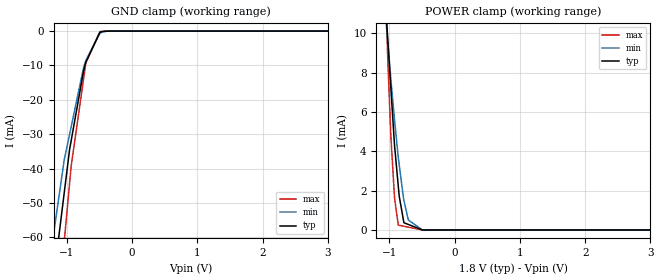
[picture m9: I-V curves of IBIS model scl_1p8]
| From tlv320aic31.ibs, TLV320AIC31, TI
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|   scl_1p8 Model
[Model]   scl_1p8
Model_type   Input
Vinl = 0.54
Vinh = 1.26
|   typ   min   max
|   (nom PVT)   (fast PVT)   (slow PVT)
|C_comp from frequency sweep method (F=400KHz)
|Average
|C_comp   2.312e-11   2.229e-11   2.341e-11
|C_comp from LC tank measurement(L=1nH)
|Average
|Resonant Frequency(Hz)   2.030e+09   2.040e+09   2.020e+09
C_comp   6.153e-12   6.093e-12   6.214e-12
| Where nom  PVT is Nominal Process, 1.8V, 26C
|   Fast PVT is Strong Process,  1.98V, -40C
|   Slow PVT is Weak Process,   1.62V, 86C
[Model Spec]
|Subparameter   typ   min   max
Vinl   0.54   0.486   0.594
Vinh   1.26   1.134   1.386
[Voltage Range]   1.8   1.62   1.98
|Ambient Temperature   25   85   -40
|Junction Temperature
[Temperature Range]   26   86   -40
[Power Clamp Reference]   1.8   1.62   1.98
[GND Clamp Reference]   0   0   0
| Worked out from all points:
|   GND clamp passes 1 mA (typ) near -0.51 V on its own axis
|   POWER clamp passes 1 mA (typ) near -0.81 V on its own axis
[GND Clamp]
|   Voltage   I(typ)   I(min)   I(max)
-1.8V     -330.6mA   -175mA     -470.5mA
-1.202V   -71.76mA   -58.79mA   -94.27mA
-1.04V    -46.94mA   -37.39mA   -61.03mA
-957.6mV  -34.34mA   -29.93mA   -44.11mA
-932.6mV  -31.68mA   -27.67mA   -39.04mA
-745.2mV  -11.71mA   -10.72mA   -14.06mA
-712.8mV  -9.192mA   -8.64mA    -9.745mA
-704.9mV  -8.873mA   -8.35mA    -9.025mA
-495mV    -409.6uA   -657.6uA   -178.1uA
-424.4mV  -70.4uA    -146.2uA   -21.27uA
-306.2mV  -3.142uA   -7.691uA   -346.8nA
3.6V      0A         0A         0A
[POWER Clamp]
|   Voltage   I(typ)   I(min)   I(max)
-1.8V     58.58mA    42.75mA    96.1mA
-1.073V   12.51mA    11.5mA     13.37mA
-1.033V   10.12mA    9.9mA      9.534mA
-1.022V   9.52mA     9.438mA    8.427mA
-976.1mV  7.154mA    7.627mA    4.701mA
-920.7mV  4.294mA    5.584mA    1.615mA
-863.3mV  2.217mA    3.671mA    247uA
-849.6mV  1.724mA    3.318mA    237.9uA
-777.6mV  369.1uA    1.512mA    189.6uA
-709.6mV  280.2uA    505.5uA    143.9uA
-494.1mV  18.69nA    1.306uA    0A
3.6V      0A         0A         0A
